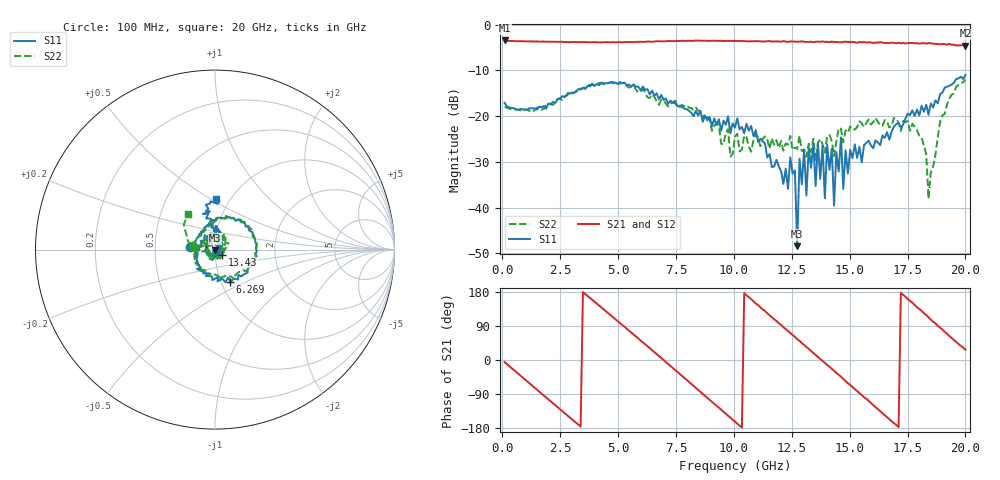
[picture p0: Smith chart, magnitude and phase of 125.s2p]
!Agilent Technologies,N5230C,MY49001569,A.09.33.09
!Agilent N5230C: A.09.33.09
!Date: Monday, July 27, 2015 15:33:44
!Correction: S11(Full 2 Port(1,2))
!S21(Full 2 Port(1,2))
!S12(Full 2 Port(1,2))
!S22(Full 2 Port(1,2))
!S2P File: Measurements: S11, S21, S12, S22:
# Hz S  dB  R 50
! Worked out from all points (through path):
!   201 points, 100 MHz to 20 GHz, reference 50 ohm
!   highest |S21| = -3.44 dB at 100 MHz (marker M1); lowest = -4.6 dB at 20 GHz (marker M2)
!   group delay of S21, straight-line fit = 146 ps
!   lowest |S11| = -48.5 dB at 12.74 GHz (marker M3), VSWR 1.01, Z = 49.9 - j0.372 ohm
!   |S11| at or under -10 dB: start of sweep to end of sweep
!   |S22| runs from -38.1 to -12.0 dB; largest |S21 - S12| = 0.024
!   S11 on the Smith chart (normalised r, x): 100 MHz: 0.76, +0.03; 6.269 GHz: 1.11, -0.41; 13.43 GHz: 1.08, -0.06; 20 GHz: 0.87, +0.53
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1e8  -17.10 173.3  -3.44 -5.7  -3.41 -5.8  -17.96 170.9
1.7915e9  -17.78 119.9  -3.68 -93.6  -3.69 -93.9  -18.35 118.4
3.483e9  -13.76 60.3  -3.80 179.2  -3.85 178.9  -13.92 59.6
6.269e9  -14.11 -64.5  -3.70 36.5  -3.69 35.8  -15.90 -63.8
6.7665e9  -16.32 -82.9  -3.64 10.4  -3.61 10.0  -17.54 -99.2
8.5575e9  -18.82 -170.6  -3.52 -84.1  -3.49 -84.1  -19.17 -175.8
1.005e10  -22.50 123.9  -3.57 -162.6  -3.57 -163.2  -24.48 66.0
1.2438e10  -29.01 34.0  -3.65 71.1  -3.73 70.6  -24.33 -107.7
1.2637e10  -31.87 32.6  -3.69 61.1  -3.80 60.5  -26.85 -120.1
1.27365e10  -48.46 -99.8  -3.74 55.0  -3.67 55.2  -27.19 -126.8
1.2836e10  -29.31 12.5  -3.71 50.3  -3.63 49.5  -24.32 -119.1
1.31345e10  -37.38 -62.3  -3.76 34.4  -3.70 34.7  -28.90 -153.8
1.3433e10  -26.07 -33.6  -3.82 18.6  -3.65 18.5  -24.97 -142.1
1.39305e10  -37.99 -52.3  -3.76 -7.6  -3.76 -7.5  -28.00 170.7
1.4229e10  -27.17 -90.8  -3.68 -23.4  -3.69 -24.2  -25.51 166.6
1.43285e10  -39.56 -158.4  -3.78 -28.4  -3.70 -29.1  -28.74 141.8
1.4627e10  -24.64 -102.0  -3.85 -44.0  -3.74 -45.4  -22.77 148.5
1.47265e10  -35.96 -99.6  -3.74 -49.7  -3.77 -50.4  -25.74 134.0
1.67165e10  -25.14 143.0  -3.99 -156.3  -3.91 -155.9  -22.49 66.2
1.81095e10  -17.72 86.7  -4.06 129.5  -4.24 128.2  -24.71 3.0
1.8408e10  -19.70 92.2  -4.02 112.5  -4.15 112.4  -38.09 -88.3
2e10  -11.04 88.6  -4.59 27.1  -4.61 26.2  -12.02 127.5
